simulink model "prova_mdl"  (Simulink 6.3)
settings: Solver=ode45  StartTime=0.0  StopTime=0.2  RelTol=1e-3
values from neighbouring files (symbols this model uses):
  b = 0.01    [prova.m]
  Ce = 10*N    (= 10)    [prova.m]
  Ia0 = 0    [prova.m]
  KI = 0.5    [prova.m]
  L = 2*mHenry    (= 0.002)    [prova.m]
  R = 1*Ohm    (= 1)    [prova.m]
  Ts = Tfin/2000    (= 0.0005)    [prova.m]
  Vin = 100*V    (= 100)    [prova.m]
  W0 = 0    [prova.m]
undefined symbols (not defined in the file or in its folder): Jm

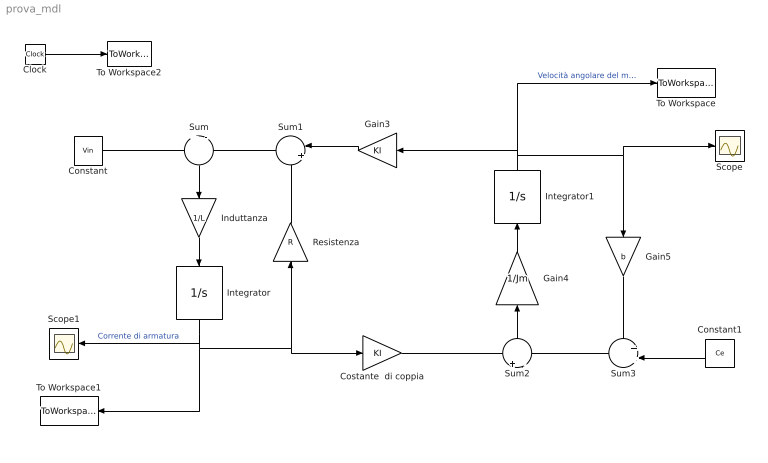
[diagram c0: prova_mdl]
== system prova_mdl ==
  Clock : Clock
  Constant : Constant  Value=Vin
  Constant1 : Constant  Orientation=left  Value=Ce
  Costante  di coppia : Gain  Gain=KI
  Gain3 : Gain  Orientation=left  Gain=KI
  Gain4 : Gain  Orientation=up  Gain=1/Jm
  Gain5 : Gain  Orientation=down  Gain=b
  Induttanza : Gain  Orientation=down  Gain=1/L
  Integrator : Integrator  Orientation=down  InitialCondition=Ia0  UpperSaturationLimit=50
  Integrator1 : Integrator  Orientation=up  InitialCondition=W0
  Resistenza : Gain  Orientation=up  Gain=R
  Scope : Scope
  Scope1 : Scope
  Sum : Sum  Orientation=down  Inputs=+|-
  Sum1 : Sum  Orientation=left  Inputs=|++
  Sum2 : Sum  Orientation=up  Inputs=+|-
  Sum3 : Sum  Orientation=left  Inputs=++|
  To Workspace : ToWorkspace  VariableName=Wm  SampleTime=Ts  SaveFormat=Array
  To Workspace1 : ToWorkspace  VariableName=Ia  SampleTime=Ts  SaveFormat=Array
  To Workspace2 : ToWorkspace  VariableName=t  SampleTime=Ts  SaveFormat=Array
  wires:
  Sum/1 -> Induttanza/1
  Induttanza/1 -> Integrator/1
  Constant/1 -> Sum/1
  Integrator/1 -> Scope1/1, Resistenza/1, Costante  di coppia/1, To Workspace1/1  "Corrente di armatura"
  Sum1/1 -> Sum/2
  Resistenza/1 -> Sum1/2
  Gain3/1 -> Sum1/1
  Costante  di coppia/1 -> Sum2/1
  Sum2/1 -> Gain4/1
  Gain4/1 -> Integrator1/1
  Integrator1/1 -> Gain3/1, Gain5/1, Scope/1, To Workspace/1  "Velocità angolare del motore"
  Sum3/1 -> Sum2/2
  Gain5/1 -> Sum3/1
  Constant1/1 -> Sum3/2
  Clock/1 -> To Workspace2/1
